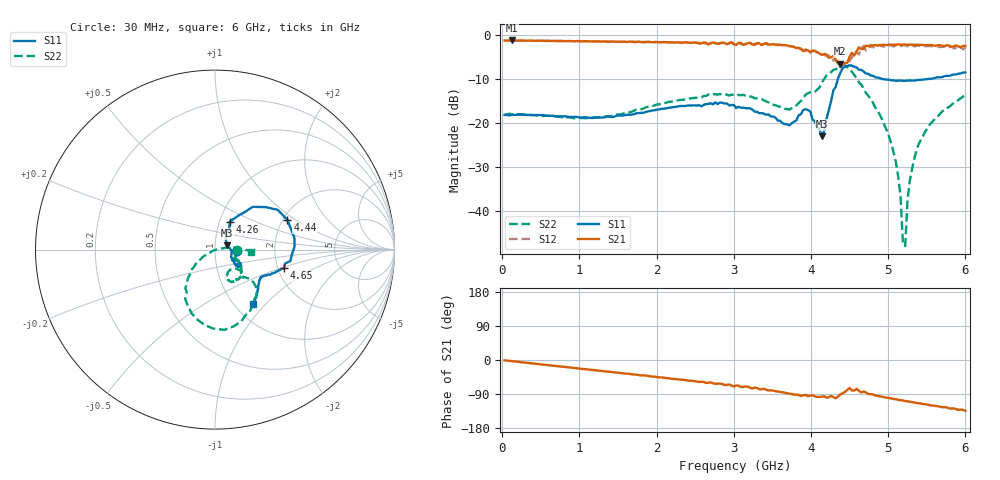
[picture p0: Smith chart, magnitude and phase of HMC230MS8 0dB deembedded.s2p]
!Hittite Microwave Corporation
!12 Elizabeth Drive
!Chelmsford, MA 01824
!Tel: 978-250-3343
!Fax: 978-250-3373
!Device: HMC230MS8, 0.75-2 GHz GaAs IC 3-bit Digital Attenuator in 8 lead plastic surface mount Mini Small Outline Package
!Misc: Room Temp Vdd = 5V , 0dB State.
# GHZ S DB R 50.0
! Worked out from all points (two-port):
!   200 points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, 30 MHz to 6 GHz, reference 50 ohm
!   highest |S21| = -1.35 dB at 120 MHz (marker M1); lowest = -6.6 dB at 4.38 GHz (marker M2)
!   |S21| within 3 dB of the highest: start of sweep to 4.115 GHz; 4.575 GHz to end of sweep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
!   lowest |S11| = -23.1 dB at 4.14 GHz (marker M3), VSWR 1.15, Z = 57 + j2.82 ohm
!   |S11| at or under -10 dB: start of sweep to 4.35 GHz; 4.909 GHz to 5.569 GHz (659.7 MHz wide, 12.6 % of centre)
!   |S22| runs from -48.0 to -6.9 dB; largest |S21 - S12| = 0.12
!   S11 on the Smith chart (normalised r, x): 30 MHz: 1.28, -0.02; 4.26 GHz: 1.12, +0.36; 4.44 GHz: 2.12, +0.86; 4.65 GHz: 2.16, -0.53; 6 GHz: 1.21, -0.85
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0.03  -18.24 -3.0  -1.36 -0.9  -1.39 -0.9  -18.23 -0.2
0.12  -18.24 -5.3  -1.35 -2.9  -1.38 -2.9  -18.06 -4.5
1.05  -18.79 -30.6  -1.55 -23.5  -1.56 -23.7  -18.96 -24.3
2.04  -16.94 -26.7  -1.78 -46.0  -1.74 -45.7  -15.82 -28.9
3.03  -16.66 -37.5  -2.37 -67.4  -2.18 -66.7  -13.87 -57.8
3.72  -20.61 -11.0  -2.64 -88.9  -2.64 -88.9  -17.05 -52.4
3.93  -16.94 -3.9  -3.41 -91.9  -3.75 -92.9  -13.64 -39.9
4.02  -19.28 -10.8  -3.70 -93.0  -3.78 -94.9  -13.19 -44.6
4.14  -23.06 20.5  -4.63 -96.7  -4.39 -98.8  -10.97 -40.4
4.26  -15.06 62.0  -5.16 -94.9  -5.12 -102.4  -8.54 -55.5
4.38  -8.68 40.0  -6.64 -90.9  -7.40 -96.5  -7.13 -76.1
4.44  -7.21 22.1  -6.50 -84.3  -6.65 -81.1  -7.14 -91.6
4.65  -8.01 -15.1  -3.33 -85.9  -3.18 -77.4  -11.35 -127.6
5.01  -10.27 -29.0  -2.32 -100.2  -2.42 -99.3  -23.09 -149.3
5.13  -10.48 -31.1  -2.26 -105.0  -2.39 -104.9  -32.28 -150.2
5.16  -10.42 -31.3  -2.32 -106.1  -2.69 -105.5  -36.78 -150.6
5.19  -10.52 -32.3  -2.30 -106.7  -2.48 -105.2  -47.02 -136.5
5.22  -10.51 -33.0  -2.27 -108.3  -2.45 -107.9  -48.01 -13.6
5.25  -10.45 -33.0  -2.34 -109.1  -2.68 -108.3  -37.63 9.1
5.28  -10.41 -34.1  -2.31 -110.0  -2.47 -108.5  -33.16 10.6
5.4  -10.29 -36.4  -2.35 -114.2  -2.52 -113.4  -24.67 10.1
6  -8.61 -55.0  -2.60 -134.5  -2.90 -128.1  -13.89 -3.8
